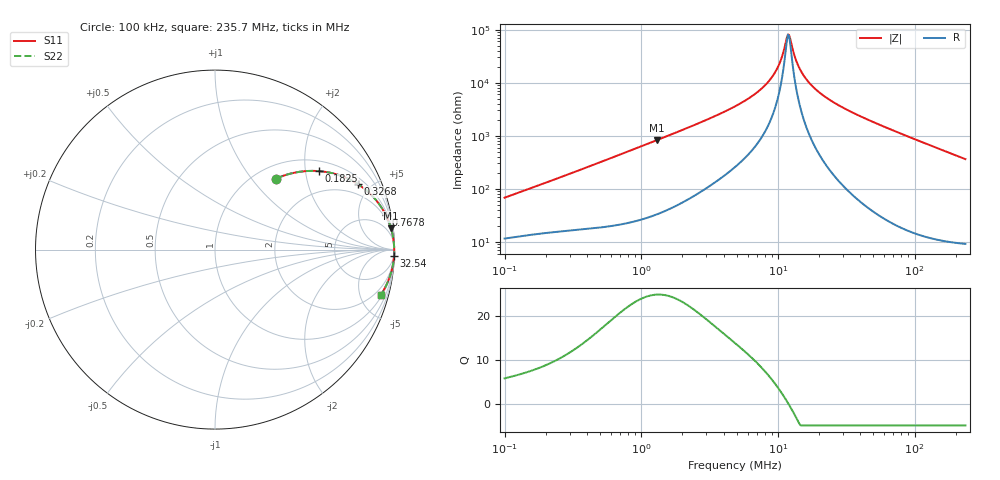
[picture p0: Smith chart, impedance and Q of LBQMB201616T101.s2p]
! LBQMB201616T101  S-PARAMETER MODEL  ( General Type )
! Model Generated by TAIYO YUDEN Corporation (http://www.ty-top.com)
! Version 1.0
! TAIYO YUDEN Control No. 191025NI43SB-FBB
! Copyright(c) 2019 TAIYO YUDEN CO.,LTD. All Rights Reserved.
! Product Description (link to TY-COMPAS)
! https://ds.yuden.co.jp/TYCOMPAS/or/detail?pn=LBQMB201616T101J&u=M
! Products Name : Inductors
! Characteristics :
!  Inductance : 100 uH , SRF(min) : 9.0 MHz , DC Resistance(max) : 10.4 Ohm , Rated Current : 80 mA
!  Case Size : 2.0 x 1.6 / 0.079 x 0.063 [mm/inch] , Thickness : 1.6 / 0.063 [mm/inch]
!  (Conditions: Temperature = 25 degC , DC Bias Current/Voltage = 0A / 0V)
! External Node Assignments :
!  1  o---GGG---o  2
! GND o---------o GND
! Frequency Range : 0.1MHz  -  235.669543MHz  [ 402 STEP ]
# MHz S RI R 50
! Freq[MHz].  S11 Real  S11 Imag  S21 Real  S21 Imag  S12 Real  S12 Imag  S22 Real  S22 Imag
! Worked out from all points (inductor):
!   401 points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, 100 kHz to 235.7 MHz, reference 50 ohm
!   read as one part in series: L = 105 uH near 104 kHz
!   highest Q = 25 at 1.297 MHz (marker M1), where L = 101 uH
!   self-resonance near 11.86 MHz
!   S11 on the Smith chart (normalised r, x): 100 kHz: 1.23, +1.34; 182.5 kHz: 1.29, +2.37; 326.8 kHz: 1.33, +4.16; 767.8 kHz: 1.44, +9.68; 32.54 MHz: 3, -60; 235.7 MHz: 1.18, -7.24
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0.1  0.3407 0.3956  0.6593 -0.3956  0.6593 -0.3956  0.3407 0.3956
0.182538  0.5782 0.4373  0.4218 -0.4373  0.4218 -0.4373  0.5782 0.4373
0.326796  0.7947 0.3659  0.2053 -0.3659  0.2053 -0.3659  0.7947 0.3659
0.367165  0.8277 0.3427  0.1723 -0.3427  0.1723 -0.3427  0.8277 0.3427
0.767767  0.951 0.1942  0.049 -0.1942  0.049 -0.1942  0.951 0.1942
1.296762  0.9808 0.1186  0.0192 -0.1186  0.0192 -0.1186  0.9808 0.1186
1.348099  0.9821 0.1142  0.0179 -0.1142  0.0179 -0.1142  0.9821 0.1142
4.854581  0.9972 0.0278  0.00278 -0.0278  0.00278 -0.0278  0.9972 0.0278
7.019984  0.9981 0.0152  0.00185 -0.0152  0.00185 -0.0152  0.9981 0.0152
8.861459  0.9985 0.0083  0.00149 -0.0083  0.00149 -0.0083  0.9985 0.0083
10.15127  0.9987 0.00448  0.00134 -0.00448  0.00134 -0.00448  0.9987 0.00448
11.62883  0.9988 0.00071  0.00123 -0.00071  0.00123 -0.00071  0.9988 0.00071
11.85678  0.9988 0.000172  0.00122 -0.000172  0.00122 -0.000172  0.9988 0.000172
12.32617  0.9988 -0.000903  0.0012 0.000903  0.0012 0.000903  0.9988 -0.000903
13.32144  0.9988 -0.00306  0.00117 0.00306  0.00117 0.00306  0.9988 -0.00306
14.39707  0.9988 -0.00525  0.00115 0.00525  0.00115 0.00525  0.9988 -0.00525
15.86456  0.9988 -0.00803  0.00115 0.00803  0.00115 0.00803  0.9988 -0.00803
17.8243  0.9988 -0.0115  0.00118 0.0115  0.00118 0.0115  0.9988 -0.0115
22.941  0.9986 -0.0196  0.00139 0.0196  0.00139 0.0196  0.9986 -0.0196
32.53614  0.9979 -0.0329  0.00209 0.0329  0.00209 0.0329  0.9979 -0.0329
65.44454  0.9932 -0.0737  0.00678 0.0737  0.00678 0.0737  0.9932 -0.0737
235.6695  0.9237 -0.2532  0.0763 0.2532  0.0763 0.2532  0.9237 -0.2532
